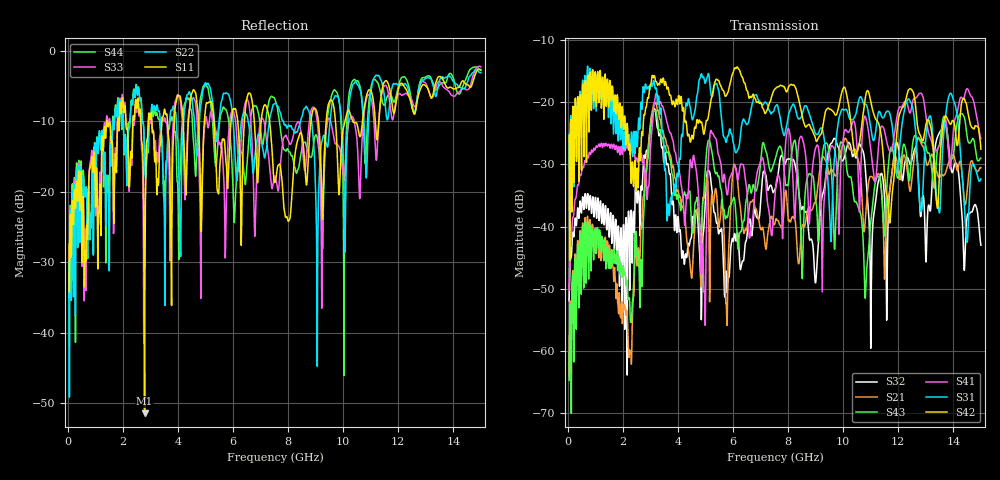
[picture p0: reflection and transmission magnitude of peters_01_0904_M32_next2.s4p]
# MHZ S RI R 50.00
! FREQ  S11  S12  S13  S14
!  S21  S22  S23  S24
!  S31  S32  S33  S34
!  S41  S42  S43  S44
!  REAL  IMAG  REAL  IMAG  REAL  IMAG  REAL  IMAG
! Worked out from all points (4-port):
!   1496 points, 50 MHz to 15 GHz, reference 50 ohm
!   strongest paths, dB at 50 MHz, 3.79 GHz, 7.53 GHz, 11.27 GHz, 15 GHz:
!     S42: -25.4, -20.3, -17.8, -23.2, -27.5
!     S31: -25.1, -35.1, -20.7, -21.8, -32.3
!     S41: -50.2, -25.8, -34.7, -27.8, -25.9
!     S43: -64.7, -31.6, -29.2, -31.9, -29.0
!     S21: -64.0, -30.4, -39.2, -31.5, -30.5
!     S32: -51.9, -36.4, -34.0, -32.9, -43.0
!   lowest |S11| = -51.4 dB at 2.79 GHz (marker M1), VSWR 1.01, Z = 50.2 - j0.223 ohm
!   |S11| at or under -10 dB: start of sweep to 1.414 GHz; 5.311 GHz to 5.931 GHz (620.7 MHz wide, 11 % of centre); 7.329 GHz to 8.83 GHz (1.501 GHz wide, 18.6 % of centre)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
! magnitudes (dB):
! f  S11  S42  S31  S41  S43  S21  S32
! 50 MHz  -27.4  -25.4  -25.1  -50.2  -64.7  -64.0  -51.9
! 760 MHz  -18.9  -22.4  -20.3  -28.7  -48.4  -45.5  -36.8
! 2.26 GHz  -17.2  -27.1  -28.2  -27.5  -53.4  -60.0  -45.3
! 2.79 GHz  -51.4  -22.0  -18.2  -31.5  -35.0  -32.9  -28.7
! 3.66 GHz  -12.2  -18.0  -36.5  -24.3  -28.1  -27.7  -30.5
! 4.94 GHz  -11.3  -25.2  -16.0  -49.6  -35.0  -35.5  -40.3
! 15 GHz  -2.7  -27.5  -32.3  -25.9  -29.0  -30.5  -43.0
